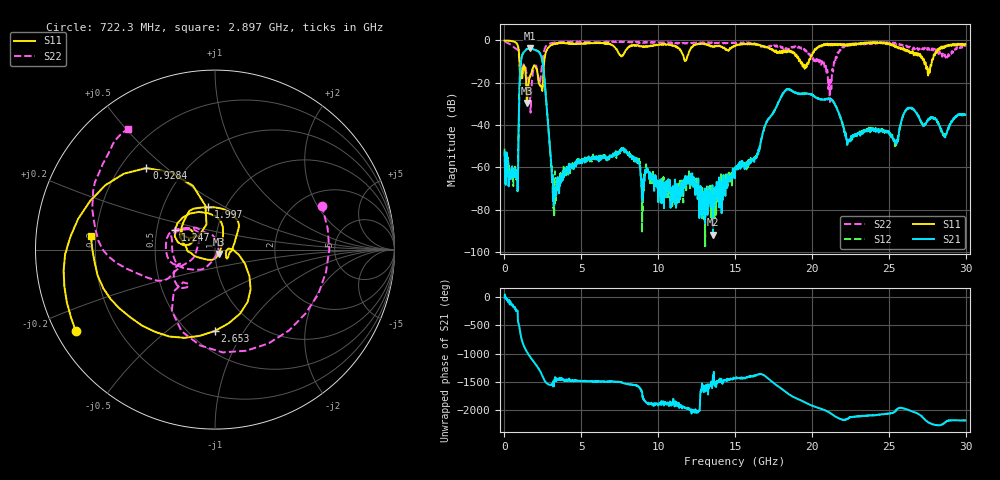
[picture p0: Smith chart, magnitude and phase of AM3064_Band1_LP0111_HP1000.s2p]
# Hz S DB R 50.0
!freq dBS11 angS11 dBS21 angS21 dBS12 angS12 dBS22 angS22
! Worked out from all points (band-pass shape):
!   1600 points, 10 MHz to 29.98 GHz, reference 50 ohm
!   highest |S21| = -3.83 dB at 1.678 GHz (marker M1); lowest = -91.8 dB at 13.56 GHz (marker M2)
!   |S21| within 3 dB of the highest: 1.163 GHz to 2.355 GHz (1.192 GHz wide, 67.8 % of centre)
!   lowest |S11| = -29.6 dB at 1.472 GHz (marker M3), VSWR 1.07, Z = 52.2 - j2.59 ohm
!   |S11| at or under -10 dB: 973.8 MHz to 2.586 GHz (1.612 GHz wide, 90.6 % of centre); 19.25 GHz to 19.8 GHz (545.2 MHz wide, 2.79 % of centre); 27.3 GHz to 27.8 GHz (494.8 MHz wide, 1.8 % of centre)
!   |S22| runs from -34.2 to -0.3 dB; largest |S21 - S12| = 0.0092
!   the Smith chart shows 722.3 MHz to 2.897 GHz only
!   S11 on the Smith chart (normalised r, x): 722.3 MHz: 0.06, -0.27; 928.4 MHz: 0.31, +0.43; 1.247 GHz: 0.62, +0.15; 1.997 GHz: 0.83, +0.42; 2.653 GHz: 0.66, -0.75; 2.897 GHz: 0.18, +0.05
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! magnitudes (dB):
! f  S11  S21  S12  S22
! 10 MHz  -0.1  -53.0  -51.2  -0.3
! 722.3 MHz  -0.9  -64.3  -63.9  -3.8
! 928.4 MHz  -4.5  -39.1  -39.1  -6.2
! 1.247 GHz  -12.1  -5.7  -5.7  -11.4
! 1.472 GHz  -29.6  -4.1  -4.1  -16.0
! 1.678 GHz  -16.6  -3.8  -3.8  -29.8
! 1.997 GHz  -12.4  -4.5  -4.5  -12.3
! 2.653 GHz  -6.9  -22.7  -22.7  -3.4
! 2.897 GHz  -3.1  -44.8  -44.7  -1.6
! 3.29 GHz  -1.7  -69.4  -61.8  -1.0
! 5.015 GHz  -1.5  -57.7  -56.3  -0.6
! 7.751 GHz  -6.6  -51.4  -51.1  -0.7
! 10 GHz  -2.1  -76.4  -67.4  -0.9
! 13.56 GHz  -2.9  -91.8  -70.2  -1.2
! 15 GHz  -2.6  -61.4  -61.6  -1.3
! 18.25 GHz  -5.0  -23.8  -23.9  -4.3
! 19.99 GHz  -7.3  -25.8  -25.7  -7.9
! 21.17 GHz  -1.9  -27.8  -27.5  -29.1
! 22.37 GHz  -2.2  -47.2  -47.9  -2.0
! 25 GHz  -1.4  -43.6  -43.5  -1.2
! 27.58 GHz  -14.6  -37.5  -37.0  -3.6
! 29.98 GHz  -1.7  -35.1  -35.3  -2.9
